| TEXAS INSTRUMENTS INCORPORATED
| Standard Linear and Logic Group
| IBIS Model of SN74AVC16245
| 16-BIT BUS TRANSCEIVER WITH 3-STATE OUTPUTS
| This file contains package information for the following:
|  TSSOP 48-pin (DGG) package as [Component] AVC16245_DGG
|  TVSOP 48-pin (DGV) package as [Component] AVC16245_DGV
| This device can be powered at the following Vccs:
|  1.2 volt Vcc
|  1.5 volt Vcc
|  1.8 volt Vcc
|  2.5 volt Vcc
|  3.3 volt Vcc
| This file provides unique models under the [Model Selector] for each Vcc.
| For operation at a specific Vcc, select the appropriate model after each
| [Model Selector] keyword.
[IBIS Ver]   3.2
[Comment char]  |_char
[File Name]   sn74avc16245.ibs
[File Rev]   1.1 | a_die
[Date]   May 29, 2003
[Source]   Data created from TI-SPICE simulations at TI-SLL.
[Notes]   The following is an IBIS list for the AVC16245.
   Please contact sllibis@ti.com with questions and
   comments concerning SLL IBIS models.
   -Power clamp data deleted as there is no power-clamp diode.
[Disclaimer] Property of Texas Instruments Incorporated.  Unauthorized
   reproduction and/or distribution is strictly prohibited.
   This product is protected under copyright law.
   Created  2003, (C) Copyright  2003, Texas Instruments
   Incorporated, All Rights Reserved
   UNLESS THERE IS A SIGNED, WRITTEN AGREEMENT TO THE
   CONTRARY, TEXAS INSTRUMENTS (TI) IS PROVIDING THE IBIS
   MODELS  AND WITHOUT ANY WARRANTY, EXPRESSED OR
   IMPLIED.  TI assumes no liability for:
   1) the accuracy of the IBIS models provided to your
   company;
   2) the proper functioning of these IBIS Models in your
   design or for any resulting applications; or
   3) infringement of patents, copyrights or intellectual
   property rights resulting from your use of these IBIS
   models.
   TI provides IBIS Models as a service to our customers.
   You and your company shall not distribute, sell or give
   these models to anyone else without prior written
   permission from TI.
   TI reserves the right to make changes to our products or
   to discontinue any semiconductor product or service
   without notice, and advises our customers to obtain the
   latest version of relevant information to verify, before
   placing orders, that the information being relied on is
   current.
   Please be aware that your receipt and use of the IBIS
   information provided shall serve as acceptance of these
   terms and conditions.  If you do not accept these terms,
   you should return or destroy the IBIS models and any
   other accompanying information immediately.
| Component AVC16245_DGG 48-pin TSSOP
[Component]   AVC16245_DGG
[Manufacturer]   Texas Instruments, Inc.
[Package]
|   typ   min   max
R_pkg   4.400e-02   3.800e-02   5.100e-02
L_pkg   3.019e-09   2.486e-09   4.099e-09
C_pkg   5.070e-13   3.340e-13   8.090e-13
[Pin]   signal_name   model_name   R_pin   L_pin   C_pin
1   1DIR   AVC16245_DIR   4.100e-02   4.017e-09   7.590e-13
2   1B1   AVC16245_IO   4.200e-02   3.737e-09   7.920e-13
3   1B2   AVC16245_IO   4.200e-02   3.480e-09   6.610e-13
4   GND   GND   3.800e-02   3.131e-09   5.750e-13
5   1B3   AVC16245_IO   4.700e-02   3.122e-09   5.660e-13
6   1B4   AVC16245_IO   4.300e-02   2.948e-09   5.040e-13
7   VCC   POWER   4.500e-02   2.845e-09   3.970e-13
8   1B5   AVC16245_IO   4.900e-02   2.835e-09   3.940e-13
9   1B6   AVC16245_IO   4.800e-02   2.715e-09   3.780e-13
10   GND   GND   5.000e-02   2.664e-09   3.630e-13
11   1B7   AVC16245_IO   5.000e-02   2.585e-09   3.480e-13
12   1B8   AVC16245_IO   4.900e-02   2.550e-09   3.370e-13
13   2B1   AVC16245_IO   4.900e-02   2.541e-09   3.360e-13
14   2B2   AVC16245_IO   5.000e-02   2.574e-09   3.480e-13
15   GND   GND   4.900e-02   2.618e-09   3.590e-13
16   2B3   AVC16245_IO   4.600e-02   2.671e-09   3.750e-13
17   2B4   AVC16245_IO   4.500e-02   2.754e-09   3.890e-13
18   VCC   POWER   4.400e-02   2.823e-09   4.500e-13
19   2B5   AVC16245_IO   4.200e-02   2.968e-09   5.030e-13
20   2B6   AVC16245_IO   5.100e-02   3.108e-09   5.350e-13
21   GND   GND   4.200e-02   3.175e-09   5.870e-13
22   2B7   AVC16245_IO   4.100e-02   3.449e-09   6.780e-13
23   2B8   AVC16245_IO   4.400e-02   3.766e-09   8.040e-13
24   2DIR   AVC16245_DIR   4.300e-02   4.065e-09   7.610e-13
25   2NOE   AVC16245_OE   4.100e-02   3.994e-09   7.570e-13
26   2A8   AVC16245_IO   3.900e-02   3.649e-09   7.890e-13
27   2A7   AVC16245_IO   3.800e-02   3.362e-09   6.600e-13
28   GND   GND   3.800e-02   3.082e-09   5.740e-13
29   2A6   AVC16245_IO   4.400e-02   2.990e-09   5.220e-13
30   2A5   AVC16245_IO   4.100e-02   2.917e-09   4.950e-13
31   VCC   POWER   4.300e-02   2.820e-09   4.480e-13
32   2A4   AVC16245_IO   4.300e-02   2.699e-09   3.850e-13
33   2A3   AVC16245_IO   4.500e-02   2.628e-09   3.720e-13
34   GND   GND   4.600e-02   2.556e-09   3.560e-13
35   2A2   AVC16245_IO   4.600e-02   2.495e-09   3.440e-13
36   2A1   AVC16245_IO   4.700e-02   2.487e-09   3.340e-13
37   1A8   AVC16245_IO   4.700e-02   2.490e-09   3.350e-13
38   1A7   AVC16245_IO   4.600e-02   2.486e-09   3.430e-13
39   GND   GND   4.500e-02   2.566e-09   3.560e-13
40   1A6   AVC16245_IO   4.400e-02   2.639e-09   3.740e-13
41   1A5   AVC16245_IO   4.300e-02   2.701e-09   3.860e-13
42   VCC   POWER   4.300e-02   2.817e-09   4.500e-13
43   1A4   AVC16245_IO   4.100e-02   2.935e-09   5.010e-13
44   1A3   AVC16245_IO   4.700e-02   3.035e-09   5.290e-13
45   GND   GND   4.300e-02   3.171e-09   5.890e-13
46   1A2   AVC16245_IO   4.000e-02   3.415e-09   6.820e-13
47   1A1   AVC16245_IO   4.300e-02   3.741e-09   8.090e-13
48   1OE   AVC16245_OE   4.400e-02   4.099e-09   7.640e-13
| Component AVC16245_DGV 48-pin TVSOP
[Component]   AVC16245_DGV
[Manufacturer]   Texas Instruments, Inc.
[Package]
|   typ   min   max
R_pkg   7.000e-02   4.900e-02   8.500e-02
L_pkg   3.013e-09   2.743e-09   3.408e-09
C_pkg   3.710e-13   2.940e-13   5.110e-13
[Pin]   signal_name   model_name   R_pin   L_pin   C_pin
1   1DIR   AVC16245_DIR   4.900e-02   3.393e-09   4.970e-13
2   1B1   AVC16245_IO   6.000e-02   3.250e-09   5.020e-13
3   1B2   AVC16245_IO   7.700e-02   3.310e-09   4.510e-13
4   GND   GND   8.500e-02   3.299e-09   4.040e-13
5   1B3   AVC16245_IO   8.300e-02   3.136e-09   3.600e-13
6   1B4   AVC16245_IO   7.700e-02   3.019e-09   3.630e-13
7   VCC   POWER   6.500e-02   2.882e-09   3.490e-13
8   1B5   AVC16245_IO   6.600e-02   2.829e-09   3.140e-13
9   1B6   AVC16245_IO   6.700e-02   2.796e-09   3.140e-13
10   GND   GND   6.900e-02   2.754e-09   3.080e-13
11   1B7   AVC16245_IO   7.000e-02   2.753e-09   3.010e-13
12   1B8   AVC16245_IO   7.100e-02   2.745e-09   2.940e-13
13   2B1   AVC16245_IO   7.000e-02   2.744e-09   2.940e-13
14   2B2   AVC16245_IO   7.000e-02   2.754e-09   3.010e-13
15   GND   GND   6.900e-02   2.754e-09   3.080e-13
16   2B3   AVC16245_IO   6.700e-02   2.796e-09   3.140e-13
17   2B4   AVC16245_IO   6.600e-02   2.829e-09   3.140e-13
18   VCC   POWER   6.500e-02   2.883e-09   3.500e-13
19   2B5   AVC16245_IO   7.500e-02   3.014e-09   3.630e-13
20   2B6   AVC16245_IO   8.000e-02   3.128e-09   3.580e-13
21   GND   GND   8.400e-02   3.295e-09   4.030e-13
22   2B7   AVC16245_IO   7.800e-02   3.311e-09   4.520e-13
23   2B8   AVC16245_IO   6.200e-02   3.259e-09   5.010e-13
24   2DIR   AVC16245_DIR   5.200e-02   3.404e-09   4.960e-13
25   2NOE   AVC16245_OE   5.300e-02   3.397e-09   5.050e-13
26   2A8   AVC16245_IO   6.200e-02   3.249e-09   5.110e-13
27   2A7   AVC16245_IO   7.700e-02   3.308e-09   4.530e-13
28   GND   GND   8.200e-02   3.289e-09   4.030e-13
29   2A6   AVC16245_IO   7.800e-02   3.121e-09   3.590e-13
30   2A5   AVC16245_IO   7.400e-02   3.010e-09   3.630e-13
31   VCC   POWER   6.500e-02   2.883e-09   3.490e-13
32   2A4   AVC16245_IO   6.700e-02   2.829e-09   3.140e-13
33   2A3   AVC16245_IO   6.700e-02   2.795e-09   3.140e-13
34   GND   GND   6.900e-02   2.753e-09   3.070e-13
35   2A2   AVC16245_IO   7.000e-02   2.753e-09   3.010e-13
36   2A1   AVC16245_IO   7.000e-02   2.743e-09   2.940e-13
37   1A8   AVC16245_IO   7.000e-02   2.743e-09   2.940e-13
38   1A7   AVC16245_IO   7.000e-02   2.753e-09   3.010e-13
39   GND   GND   6.900e-02   2.754e-09   3.070e-13
40   1A6   AVC16245_IO   6.800e-02   2.797e-09   3.140e-13
41   1A5   AVC16245_IO   6.700e-02   2.830e-09   3.140e-13
42   VCC   POWER   6.400e-02   2.880e-09   3.490e-13
43   1A4   AVC16245_IO   7.200e-02   3.004e-09   3.620e-13
44   1A3   AVC16245_IO   7.800e-02   3.121e-09   3.590e-13
45   GND   GND   8.400e-02   3.296e-09   4.030e-13
46   1A2   AVC16245_IO   7.700e-02   3.308e-09   4.510e-13
47   1A1   AVC16245_IO   6.200e-02   3.258e-09   4.990e-13
48   1OE   AVC16245_OE   5.300e-02   3.408e-09   4.940e-13
| Model AVC16245_DIR
[Model Selector]   AVC16245_DIR
AVC16245_DIR_12A   1.2 volt Vcc
AVC16245_DIR_15A   1.5 volt Vcc
AVC16245_DIR_18   1.8 volt Vcc
AVC16245_DIR_25   2.5 volt Vcc
AVC16245_DIR_33   3.3 volt Vcc
| Model AVC16245_OE
[Model Selector]   AVC16245_OE
AVC16245_OE_12A   1.2 volt Vcc
AVC16245_OE_15A   1.5 volt Vcc
AVC16245_OE_18   1.8 volt Vcc
AVC16245_OE_25   2.5 volt Vcc
AVC16245_OE_33   3.3 volt Vcc
| Model AVC16245_IO
[Model Selector]   AVC16245_IO
AVC16245_IO_12A   1.2 volt Vcc
AVC16245_IO_15A   1.5 volt Vcc
AVC16245_IO_18   1.8 volt Vcc
AVC16245_IO_25   2.5 volt Vcc
AVC16245_IO_33   3.3 volt Vcc
| Models and submodels in the file (15): AVC16245_DIR_12A (Input), AVC16245_DIR_15A (Input), AVC16245_DIR_18 (Input), AVC16245_DIR_25 (Input), AVC16245_DIR_33 (Input), AVC16245_OE_12A (Input), AVC16245_OE_15A (Input), AVC16245_OE_18 (Input), AVC16245_OE_25 (Input), AVC16245_OE_33 (Input), AVC16245_IO_12A (I/O), AVC16245_IO_15A (I/O), AVC16245_IO_18 (I/O), AVC16245_IO_25 (I/O), AVC16245_IO_33 (I/O)
